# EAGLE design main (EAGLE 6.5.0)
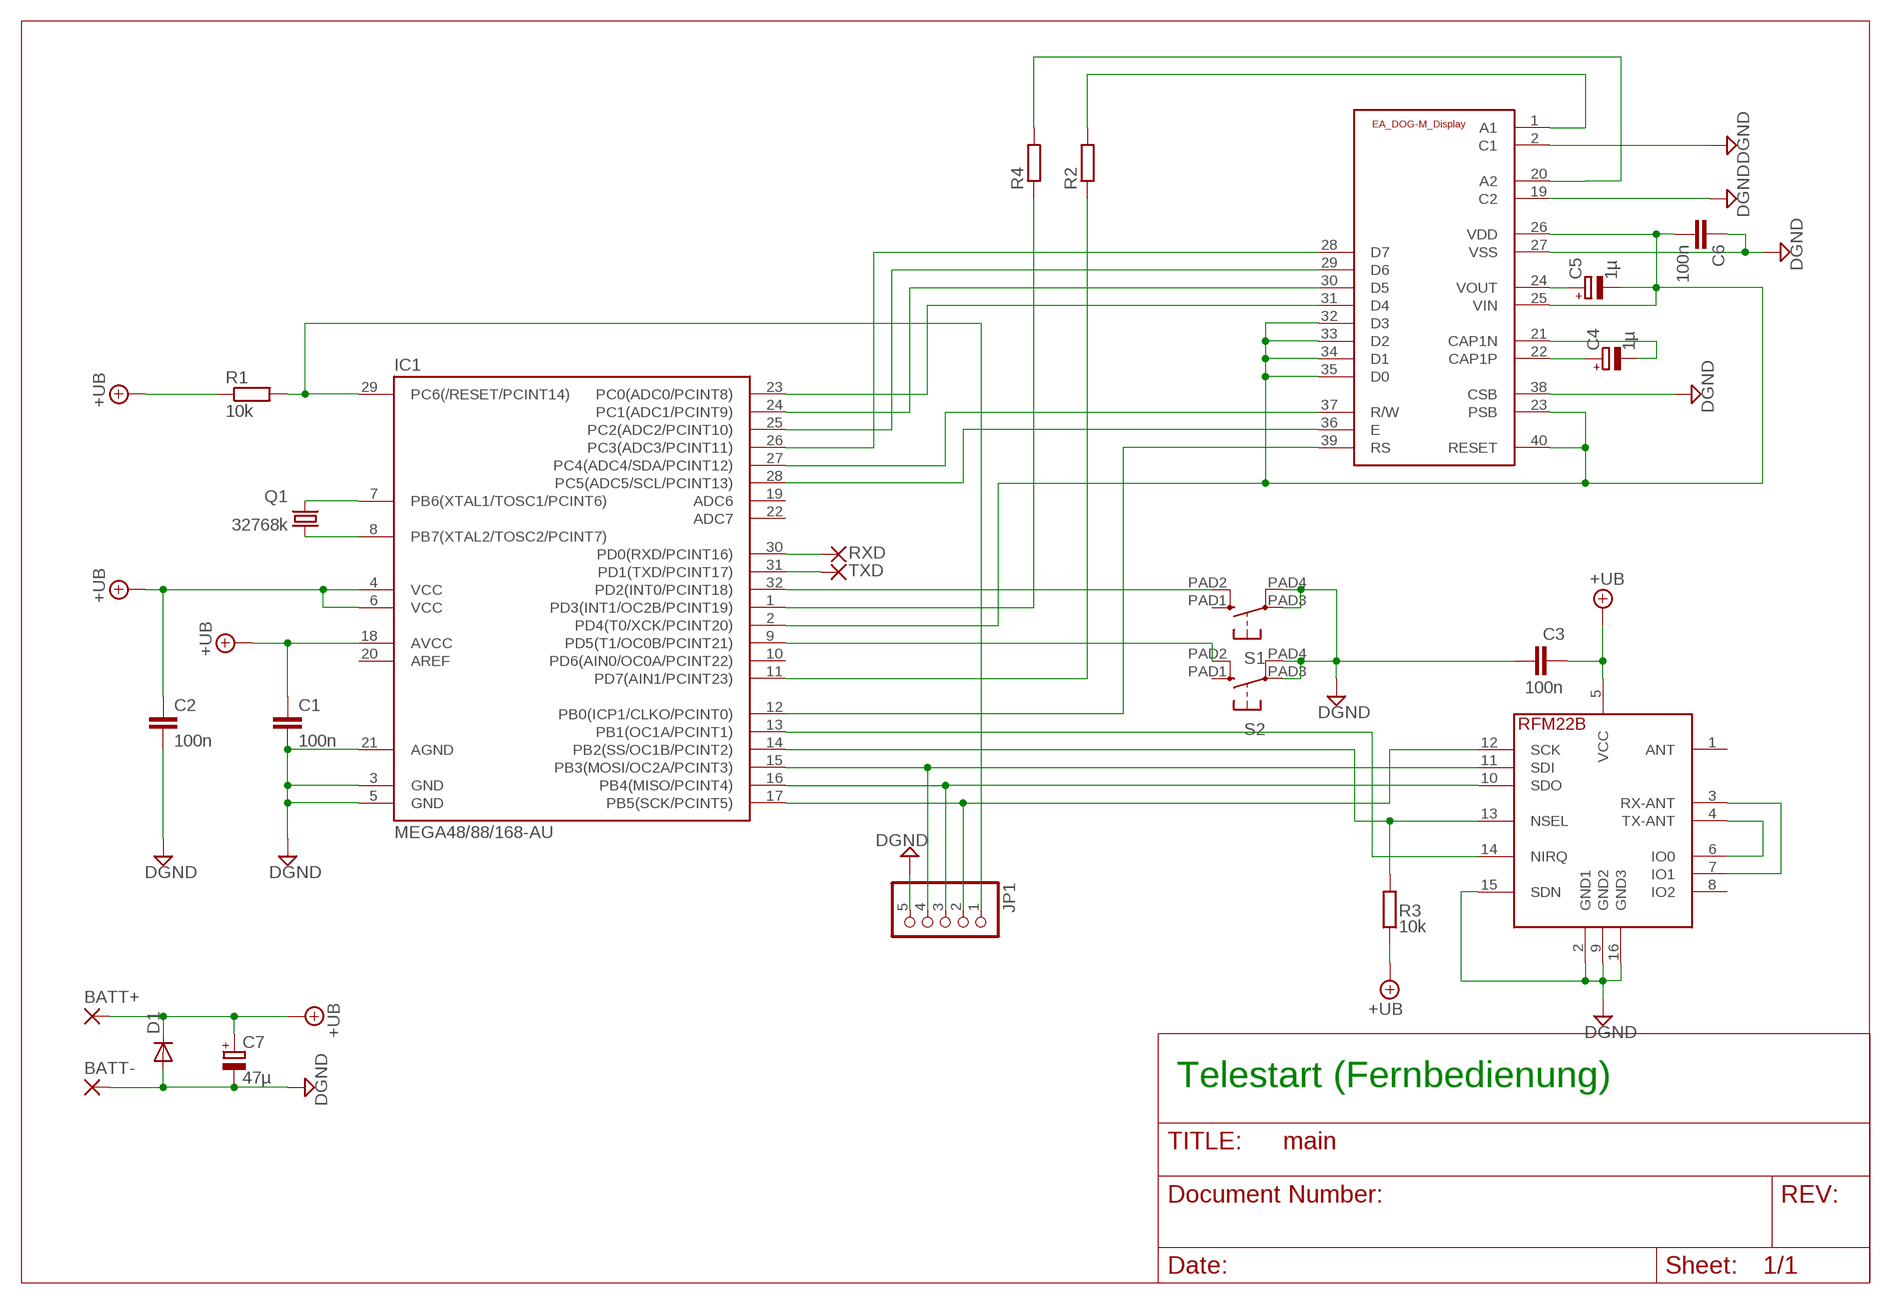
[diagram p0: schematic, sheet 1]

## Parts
BATT+  SMD2  [SMD1,27-2,54]
BATT-  SMD2  [SMD1,27-2,54]
C1  100n  C-EUC0805  [C0805]
C2  100n  C-EUC0805  [C0805]
C3  100n  C-EUC0805  [C0805]
C4  1µ  CPOL-EUSMCB  [SMC_B]
C5  1µ  CPOL-EUSMCB  [SMC_B]
C6  100n  C-EUC0805  [C0805]
C7  47µ  CPOL-EUD  [PANASONIC_D]
D1  DIODE-DO-214AC  [DO-214AC]
IC1  MEGA48/88/168-AU  [TQFP32-08]
JP1  PINHD-1X5  [1X05]
Q1  32768k  CRYSTALTC26H  [TC26H]
R1  10k  R-EU_M1206  [M1206]
R2  R-EU_M1206  [M1206]
R3  10k  R-EU_M1206  [M1206]
R4  R-EU_M1206  [M1206]
RXD  SMD2  [SMD1,27-2,54]
S1  10-XXSMD  [B3F-10_SMD]
S2  10-XXSMD  [B3F-10_SMD]
TXD  SMD2  [SMD1,27-2,54]
U$1  EA_DOG-M_DISPLAY  [E_DOG-M_DISPLAY]
U$2  RFM22B_SMD  [RFM_16PIN_SMD]

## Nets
+UB: BATT+.1(P) C1.1 C2.1 C3.2 C7.+ D1.C IC1.4(VCC) IC1.6(VCC) IC1.18(AVCC) R1.1 R3.1 U$2.5(VCC)
DGND: BATT-.1(P) C1.2 C2.2 C3.1 C6.1 C7.- D1.A IC1.3(GND) IC1.5(GND) IC1.21(AGND) JP1.5 S1.PAD3(P) S1.PAD4(P1) S2.PAD3(P) S2.PAD4(P1) U$1.2(C1) U$1.19(C2) U$1.27(VSS) U$1.38(CSB) U$2.2(GND1) U$2.9(GND2) U$2.15(SDN) U$2.16(GND3)
LED1: R2.2 U$1.1(A1)
LED2: R4.2 U$1.20(A2)
N$1: IC1.7(PB6(XTAL1/TOSC1/PCINT6)) Q1.2
N$2: IC1.8(PB7(XTAL2/TOSC2/PCINT7)) Q1.1
N$3: IC1.17(PB5(SCK/PCINT5)) JP1.2 U$2.12(SCK)
N$4: IC1.16(PB4(MISO/PCINT4)) JP1.3 U$2.10(SDO)
N$5: IC1.28(PC5(ADC5/SCL/PCINT13)) U$1.36(E)
N$6: IC1.15(PB3(MOSI/OC2A/PCINT3)) JP1.4 U$2.11(SDI)
N$7: IC1.32(PD2(INT0/PCINT18)) S1.PAD2(S1)
N$8: IC1.29(PC6(/RESET/PCINT14)) JP1.1 R1.2
N$9: IC1.11(PD7(AIN1/PCINT23)) R2.1
N$10: U$2.4(TX-ANT) U$2.6(IO0)
N$11: U$2.3(RX-ANT) U$2.7(IO1)
N$12: IC1.13(PB1(OC1A/PCINT1)) U$2.14(NIRQ)
N$13: IC1.14(PB2(SS/OC1B/PCINT2)) R3.2 U$2.13(NSEL)
N$14: IC1.23(PC0(ADC0/PCINT8)) U$1.31(D4)
N$15: IC1.24(PC1(ADC1/PCINT9)) U$1.30(D5)
N$16: IC1.25(PC2(ADC2/PCINT10)) U$1.29(D6)
N$17: IC1.26(PC3(ADC3/PCINT11)) U$1.28(D7)
N$18: IC1.9(PD5(T1/OC0B/PCINT21)) S2.PAD2(S1)
N$19: IC1.12(PB0(ICP1/CLKO/PCINT0)) U$1.39(RS)
N$20: IC1.1(PD3(INT1/OC2B/PCINT19)) R4.1
N$21: IC1.27(PC4(ADC4/SDA/PCINT12)) U$1.37(R/W)
N$22: C5.+ U$1.24(VOUT)
N$23: C4.+ U$1.22(CAP1P)
N$24: C4.- U$1.21(CAP1N)
N$25: IC1.30(PD0(RXD/PCINT16)) RXD.1(P)
N$26: IC1.31(PD1(TXD/PCINT17)) TXD.1(P)
N$31: C5.- C6.2 IC1.2(PD4(T0/XCK/PCINT20)) U$1.23(PSB) U$1.25(VIN) U$1.26(VDD) U$1.32(D3) U$1.33(D2) U$1.34(D1) U$1.35(D0) U$1.40(RESET)
Unconnected: IC1.10(PD6(AIN0/OC0A/PCINT22)) IC1.19(ADC6) IC1.20(AREF) IC1.22(ADC7) S1.PAD1(S) S2.PAD1(S) U$2.1(ANT) U$2.8(IO2)

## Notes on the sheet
- Telestart (Fernbedienung)

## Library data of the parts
BATT+ BATT- RXD TXD = wirepad:SMD2: SMD PAD
C1-C3 C6 = rcl:C-EU: CAPACITOR, European symbol
C4 C5 C7 = rcl:CPOL-EU: POLARIZED CAPACITOR, European symbol
D1 = diode:DIODE-: DIODE
IC1 = avr-4:MEGA48/88/168
JP1 = pinhead:PINHD-1X5: PIN HEADER
Q1 = crystal:CRYSTAL: CRYSTAL; OC_FARNELL: unknown; OC_NEWARK: unknown
R1-R4 = rcl:R-EU_: RESISTOR, European symbol
S1 S2 = switch-omron:10-XX: OMRON SWITCH
U$1 = display_ea_dog-m:EA_DOG-M_DISPLAY
U$2 = rfm:RFM22B_SMD

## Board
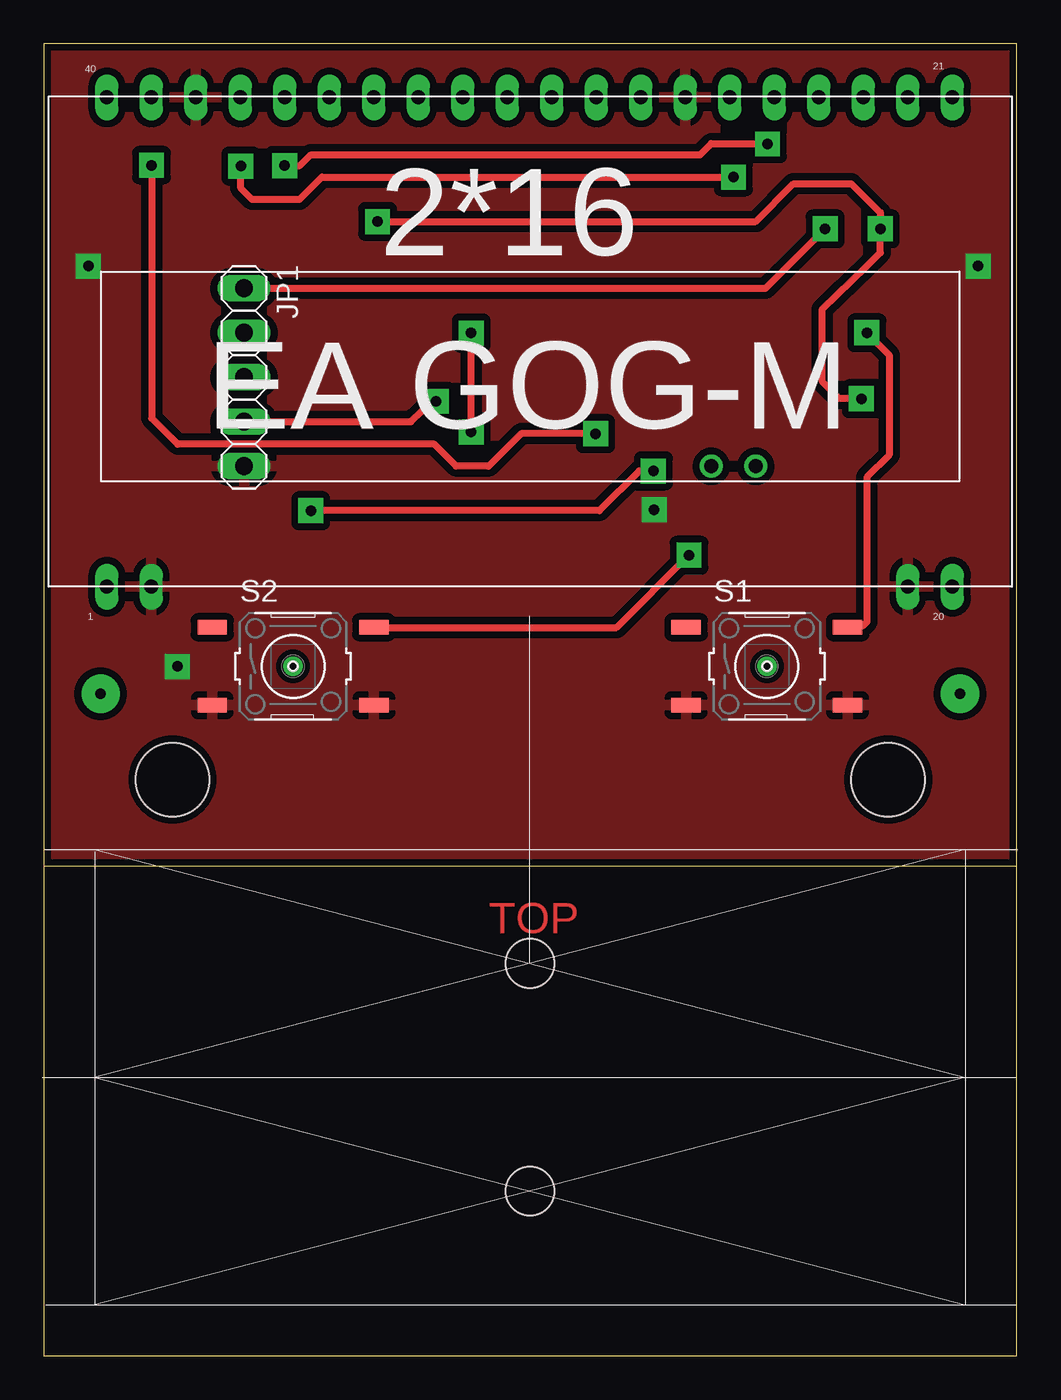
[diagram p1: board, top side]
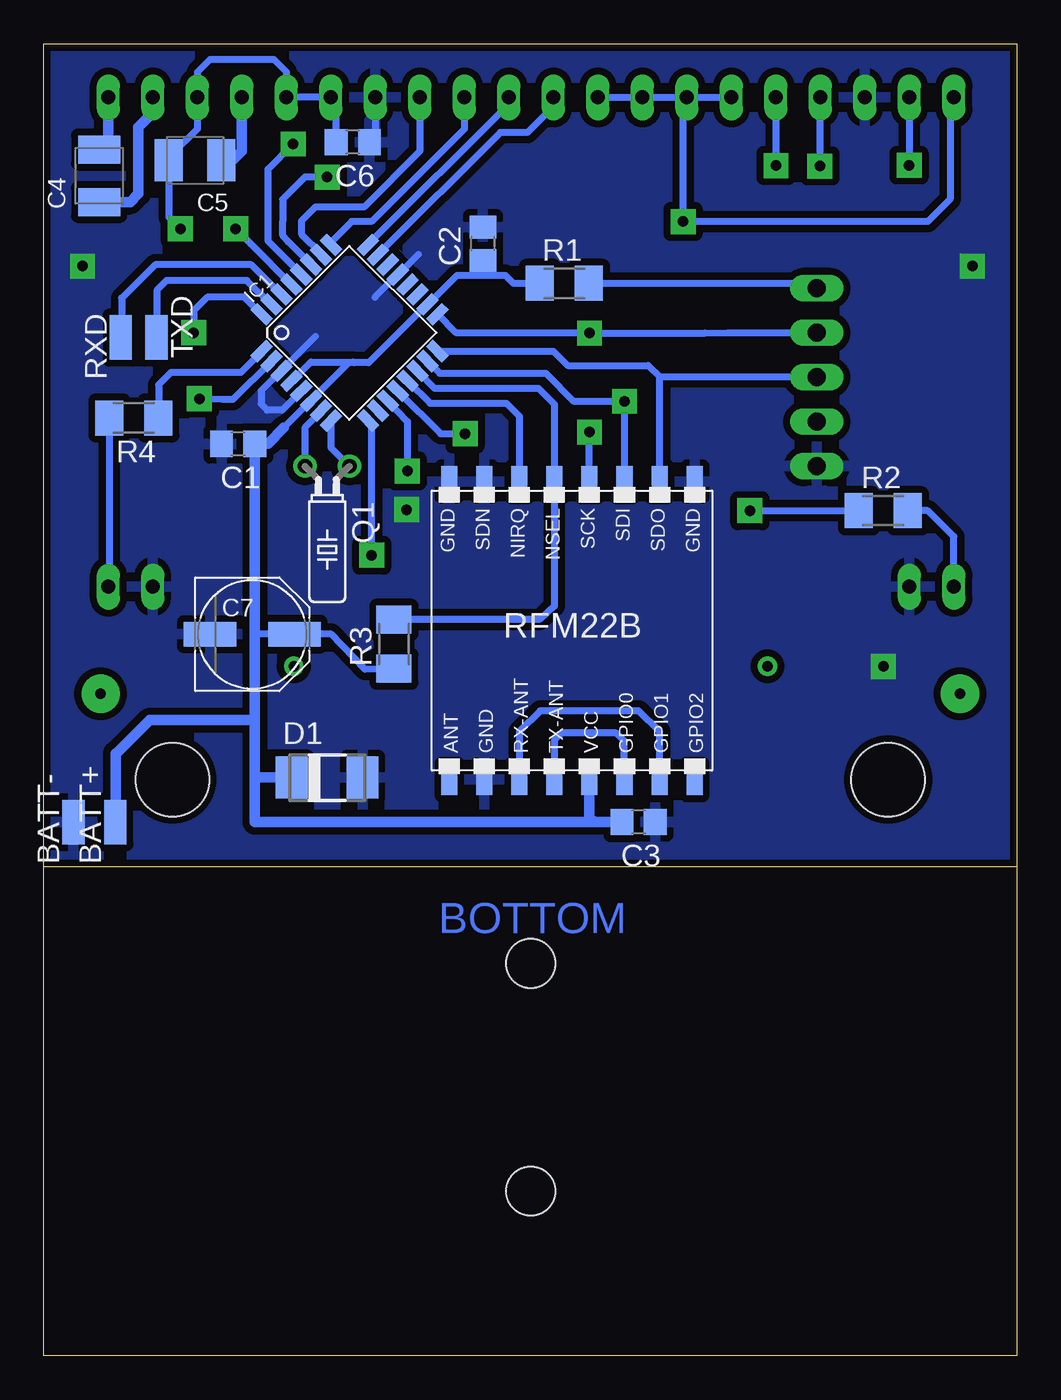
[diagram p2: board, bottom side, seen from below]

Size 55.55 x 74.92 mm. Coordinates in mm from the lower left corner, seen from the top.
Outline: 55.55,27.95 55.55,0 0,0 0,27.94
Outline: 55.55,27.95 55.55,74.92 0,74.92 0,27.94
Outline: 55.55,27.95 0,27.94
Copper layers (1*16): Top 0.035mm / dielectric 1.5mm / Bottom 0.035mm
Design rules "default": minimum track width 10mil, minimum drill 24mil, track to track 8mil, track to pad 8mil, pad to pad 8mil, via to via 8mil, smd to smd 8mil, copper to edge 4mil, drill to drill 8mil, minimum pad ring 10mil, minimum via ring 8mil, stop-mask expansion 4mil, vias tented up to drill 0mil, thermal gap 15mil
Holes 2.8 mm at 27.75,9.4 27.75,22.4
Holes 4.2 mm at 7.35,32.9 48.2,32.9

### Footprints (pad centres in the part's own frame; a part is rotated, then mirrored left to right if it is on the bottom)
SMD1,27-2,54 = smd 1.27 x 2.54: 1 0,0
C0805 = smd 1.3 x 1.5: 1 -0.95,0; 2 0.95,0
SMC_B = smd 1.6 x 2.4: + -1.5,0; - 1.5,0
PANASONIC_D = smd 3 x 1.4: + 2.4,0; - -2.4,0
DO-214AC = smd 1.8 x 2.4: A 2.025,0; C -2.025,0
TQFP32-08 = smd 1.27 x 0.559: 1 -4.293,2.8; 2 -4.293,2; 3 -4.293,1.2; 4 -4.293,0.4; 5 -4.293,-0.4; 6 -4.293,-1.2; 7 -4.293,-2; 8 -4.293,-2.8; 17 4.293,-2.8; 18 4.293,-2; 19 4.293,-1.2; 20 4.293,-0.4; 21 4.293,0.4; 22 4.293,1.2; 23 4.293,2; 24 4.293,2.8 | smd 0.559 x 1.27: 9 -2.8,-4.293; 10 -2,-4.293; 11 -1.2,-4.293; 12 -0.4,-4.293; 13 0.4,-4.293; 14 1.2,-4.293; 15 2,-4.293; 16 2.8,-4.293; 25 2.8,4.293; 26 2,4.293; 27 1.2,4.293; 28 0.4,4.293; 29 -0.4,4.293; 30 -1.2,4.293; 31 -2,4.293; 32 -2.8,4.293
1X05 = drill 1.016 long: 1 -5.08,0; 2 -2.54,0; 3 0,0; 4 2.54,0; 5 5.08,0
TC26H = drill 0.813: 1 -1.27,0; 2 1.27,0
M1206 = smd 1.6 x 2: 1 -1.4,0; 2 1.4,0
B3F-10_SMD = drill 0.6: P$1 0,0 | smd 1.676 x 0.813: PAD1 -4.61,2.223; PAD2 4.61,2.223; PAD3 -4.61,-2.223; PAD4 4.61,-2.223
E_DOG-M_DISPLAY = drill 0.8 long: 1 3.334,0; 2 5.874,0; 19 49.054,0; 20 51.594,0; 21 51.594,27.94; 22 49.054,27.94; 23 46.514,27.94; 24 43.974,27.94; 25 41.434,27.94; 26 38.894,27.94; 27 36.354,27.94; 28 33.814,27.94; 29 31.274,27.94; 30 28.734,27.94; 31 26.194,27.94; 32 23.654,27.94; 33 21.114,27.94; 34 18.574,27.94; 35 16.034,27.94; 36 13.494,27.94; 37 10.954,27.94; 38 8.414,27.94; 39 5.874,27.94; 40 3.334,27.94
RFM_16PIN_SMD = smd 1.778 x 0.914: 1 -9,7; 2 -9,5; 3 -9,3; 4 -9,1; 5 -9,-1; 6 -9,-3; 7 -9,-5; 8 -9,-7; 9 8,-7; 10 8,-5; 11 8,-3; 12 8,-1; 13 8,1; 14 8,3; 15 8,5; 16 8,7

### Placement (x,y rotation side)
BATT+  51.47,30.48 0 bottom
BATT-  53.86,30.48 0 bottom
C1  44.45,52.07 180 bottom
C2  30.48,63.5 90 bottom
C3  21.59,30.48 180 bottom
C4  52.39,67.38 90 bottom
C5  46.91,68.26 180 bottom
C6  37.91,69.3 180 bottom
C7  43.65,41.2 0 bottom
D1  39.37,33.02 0 bottom
IC1  38.1,58.42 45 bottom
JP1  11.43,55.88 270 top
Q1  39.37,50.8 180 bottom
R1  25.83,61.24 0 bottom
R2  7.62,48.26 0 bottom
R3  35.56,40.64 90 bottom
R4  50.41,53.55 180 bottom
RXD  51.15,58.15 0 bottom
S1  41.28,39.37 0 top
S2  14.23,39.37 0 top
TXD  49.11,58.15 180 bottom
U$1  0.27,43.92 0 top
U$2  25.4,41.91 90 bottom

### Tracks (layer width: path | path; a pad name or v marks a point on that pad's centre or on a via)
+UB
  Bottom 0: C1.1 43.18,52.07 43.18,52.1
  Bottom 0.406: 37.85,56.7 37,56.7 IC1.18 33.61,60.04 31.95,61.7 30.48,61.7 | 37.85,56.7 38.15,56.7 40.29,54.56 IC1.6 40.31,54.54 41.85,53 | 37.85,56.7 37.9,56.75 40.3,56.75 41.38,55.67 IC1.4 41.43,55.67 | 43.46,43.74 43.5,43.7 | 43.55,41.15 43.5,41.2 C7.+ 39.15,41.2 37.2,39.2 R3.1 | 30.48,61.7 29.2,61.7 28.75,61.25 R1.1 | C2.1 30.48,61.7
  Bottom 0.61: 24.13,30.48 43.5,30.48 43.5,33 | 24.13,30.48 C3.2 | U$2.5 24.4,30.75 24.13,30.48 | 43.18,52.1 43.5,52.1 | 43.5,36.25 43.5,41.2 43.5,43.7 C1.1 43.47,52.1 42.75,52.1 41.85,53 | 43.5,36.25 43.5,33 | D1.C 43.48,33.02 43.5,33 | BATT+.1 51.45,30.48 51.45,34.4 51.4,34.4 49.5,36.3 43.55,36.3 43.5,36.25
DGND  (via drill 0.6 pad 1.42)
  Bottom 0.406: U$1.27 36.62,69.58 36.95,69.25 C6.1 36.6,69.65 | 34.15,62.9 35.31,61.74 IC1.21 35.36,61.74 36.65,60.45 | 40.05,58.2 41.98,56.27 IC1.3 42.02,56.23 43.15,55.1 43.15,54.35 42.8,54 41.95,54 IC1.5
  other vias: 2.54,62.23 7.62,39.37 34.84,48.32 53.34,62.23
  pour Bottom (isolate 0.406): -1.27,76.2 59.69,76.2 57.15,74.93 57.15,26.67 -1.27,26.67
  pour Top (isolate 0.406): -2.54,74.93 55.88,74.93 55.88,26.67 0,26.67 -1.27,27.94 -1.27,73.66
LED1
  Bottom 0.406: U$1.1 3.6,46.78 5.08,48.26 R2.2
LED2
  Bottom 0.406: R4.2 51.81,43.97 U$1.20
N$1
  Bottom 0.406: IC1.7 39.72,53.93 40.65,53 Q1.2
N$2
  Bottom 0.406: IC1.8 39.16,51.85 Q1.1
N$3  (via drill 0.6 pad 1.42)
  Top 0.406: v24.4,52.75 v24.4,58.4 v24.4,58.41
  Bottom 0.406: U$2.12 v24.4,52.75 | IC1.17 33.1,59.49 33.1,59.5 32,58.4 v24.4,58.4 17.8,58.4 16.51,58.42 JP1.2
N$4
  Bottom 0.406: U$2.10 20.4,55.9 | JP1.3 20.32,55.88 20.34,55.9 20.4,55.9 | IC1.16 26.46,57.37 25.65,56.55 21.05,56.55 20.4,55.9
N$5  (via drill 0.6 pad 1.42)
  Top 0.406: v13.75,67.97 14.62,67.97 15.24,68.58 37.47,68.58 38.1,69.22 41.3,69.22 v41.31,69.2
  Bottom 0.406: IC1.28 40.85,61.75 42.75,63.65 42.75,67.77 v41.31,69.2 | v13.75,67.97 13.75,71.85 U$1.36
N$6  (via drill 0.6 pad 1.42)
  Top 0.406: JP1.4 20.95,53.34 22.14,54.5 v22.4,54.5
  Bottom 0.406: IC1.15 32.95,56.1 26.89,56.1 25.29,54.5 v22.4,54.5 U$2.11
N$7  (via drill 0.6 pad 1.42)
  Top 0.406: v46.99,58.42 48.26,57.15 48.26,51.44 46.99,50.16 46.99,41.91 46.77,41.69 S1.PAD2
  Bottom 0.406: IC1.32 44.1,60.45 46.23,60.45 46.99,59.69 v46.99,58.42
N$8  (via drill 0.6 pad 1.42)
  Top 0.406: v44.6,64.35 41.21,60.96 JP1.1
  Bottom 0.406: v44.6,64.35 43.75,63.5 IC1.29 | R1.2 11.71,61.24 JP1.1
N$9  (via drill 0.6 pad 1.42)
  Top 0.406: v15.24,48.26 31.71,48.26 33.98,50.53 v34.8,50.53
  Bottom 0.406: IC1.11 35.91,54.51 34.8,53.35 v34.8,50.53 | v15.24,48.26 R2.1
N$10
  Bottom 0.406: U$2.6 22.4,35.1 22.86,35.56 25.99,35.56 26.4,35.15 U$2.4
N$11
  Bottom 0.406: U$2.7 20.4,35.64 21.59,36.83 27.22,36.83 28.4,35.65 U$2.3
N$12
  Bottom 0.406: IC1.13 34.77,55.67 33.5,54.4 29.15,54.4 28.4,53.65 U$2.14 28.4,49.85
N$13
  Bottom 0.406: R3.2 27.25,42.05 26.4,42.8 U$2.13 26.4,54.34 27.31,55.25 33.25,55.25 34.22,56.22 IC1.14
N$14
  Bottom 0.406: U$1.31 26.46,71.33 27.94,69.85 29.5,69.85 IC1.23
N$15
  Bottom 0.406: U$1.30 29,71.48 IC1.24
N$16
  Bottom 0.406: U$1.29 31.54,70.06 36.83,64.77 37.98,64.77 39.15,63.6 39.15,63.46 39.16,63.45 IC1.25
N$17
  Bottom 0.406: U$1.28 34.08,68.79 37.27,65.6 40.05,65.6 40.85,64.8 40.85,64.05 39.72,62.92 IC1.26
N$18  (via drill 0.6 pad 1.42)
  Top 0.406: S2.PAD2 32.7,41.59 v36.83,45.72
  Bottom 0.406: v36.83,45.72 36.83,53.34 36.9,53.41 IC1.9
N$19  (via drill 0.6 pad 1.42)
  Top 0.406: v31.5,52.65 27.25,52.65 25.4,50.8 23.54,50.8 22.29,52.05 7.64,52.05 6.15,53.54 v6.15,67.98
  Bottom 0.406: IC1.12 32.9,52.65 v31.5,52.65 | U$1.39 v6.15,67.98
N$20
  Bottom 0: R4.1 49.53,53.55 | 49.53,53.55 49.53,53.34 | 49,53.6 49.53,53.6 49.53,53.55
  Bottom 0.406: IC1.1 43.12,57.34 44.3,56.15 48.3,56.15 49,55.45 49,53.6 49.05,53.55
N$21  (via drill 0.6 pad 1.42)
  Top 0.406: v39.37,67.31 15.88,67.31 14.61,66.04 11.88,66.04 11.25,66.67 v11.25,67.94
  Bottom 0.406: U$1.37 11.25,71.83 v11.25,67.94 | IC1.27 41.6,63.62 41.9,63.95 41.91,64.77 41.91,66.04 40.64,67.31 v39.37,67.31
N$22
  Bottom 0.61: U$1.24 44.24,68.79 44.77,68.26 C5.+
N$23
  Bottom 0.61: U$1.22 49.32,70.98 50.15,70.15 50.15,66.35 50.62,65.88 C4.+
N$24
  Bottom 0.61: U$1.21 51.86,69.41 C4.-
N$25
  Bottom 0: 51.1,58.15 RXD.1
  Bottom 0.406: IC1.30 42.01,60.61 43.7,62.3 49.2,62.3 51.1,60.4 51.1,58.15 51.15,58.1
N$26
  Bottom 0: TXD.1
  Bottom 0.406: IC1.31 42.59,60.04 43.95,61.4 48.55,61.4 49.1,60.85 TXD.1
N$27  (via drill 0.6 pad 3.81)
  other vias: 48.2,32.9
N$28  (via drill 0.6 pad 3.81)
  other vias: 7.35,32.9
N$29  (via drill 0.6 pad 2.18)
  other vias: 3.25,37.8
N$30  (via drill 0.6 pad 2.18)
  other vias: 52.3,37.8
N$31  (via drill 0.6 pad 1.42)
  Top 0.406: v46.67,54.65 45.4,54.67 44.45,55.62 44.45,59.78 46.99,62.23 47.75,62.99 v47.75,64.35 47.75,65.28 46.1,66.92 42.8,66.92 40.64,64.77 v19.05,64.77
  Bottom 0.406: IC1.2 44.75,54.6 45.35,54.6 v46.67,54.65 | v47.75,64.35 48.4,65 48.4,68.44 48.26,68.58 | 48.26,68.58 46.78,70.06 U$1.23 46.78,73.3 46.07,74.01 42.4,74.01 41.7,73.32 U$1.25 U$1.26 38.86,71.56 C6.2 | 48.26,68.58 48.26,68.41 C5.- | U$1.32 U$1.33 U$1.34 | U$1.34 U$1.35 | U$1.40 3.81,71.86 3.81,66.04 5.08,64.77 v19.05,64.77 19.05,71.65 U$1.34

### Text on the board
Top: TOP
Bottom: BOTTOM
